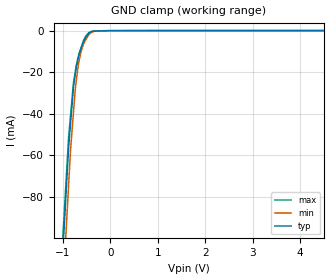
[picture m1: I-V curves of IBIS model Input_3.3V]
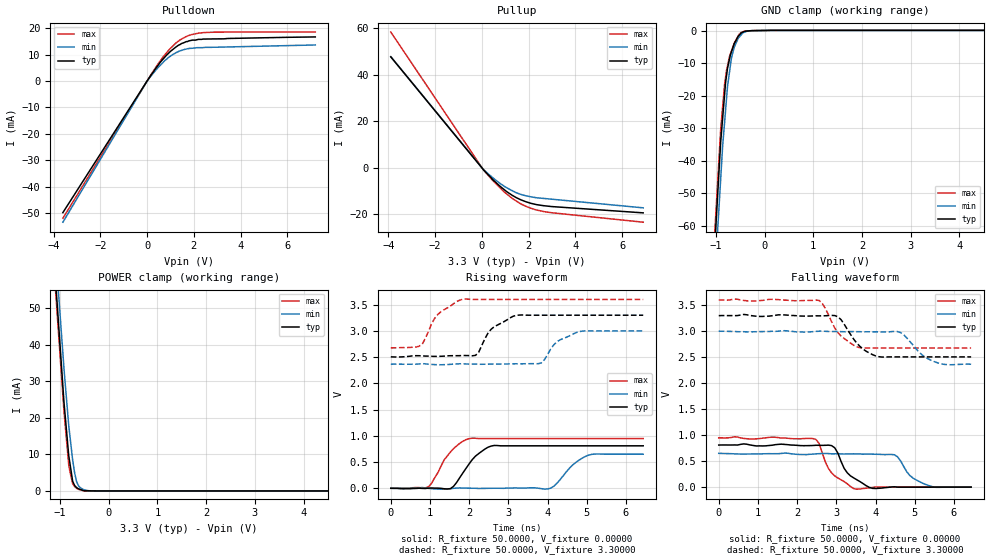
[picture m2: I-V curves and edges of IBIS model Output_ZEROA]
[IBIS Ver]   3.2
[Comment Char] |_char
[File Name]   pcm1748e.ibs
[File Rev]   3.0
[Source]
| This model file was created by Teraspeed Consulting Group LLC
| (http://www.teraspeed.com/).
[Date]   10-06-2004
[Notes]   Quality Check of this IBIS model: Model Passes IBIS Check
   Model parses into ICX IS. Simulation done with Hyperlynx.
   1. MIN TYP MAX information is based on Temprature and Voltage
   characteristics only.
[Disclaimer]
| This model is designed as an aid for customers of Texas Instruments.
| TI and its licensors and suppliers make no warranties, either expressed
| or implied, with respect to this  model, including the warranties of
| merchantability or fitness for a particular purpose.
| The model is provided solely on an "as is" basis. The entire risk as to
| its quality and performance is with the customer.
[Copyright]
| (C) Copyright 2008 Texas Instruments Incorporated. All rights reserved.
[Component] PCM1748E
[Manufacturer] TI
[Package]
| variable   typ   min   max
R_pkg  1.8006E-02  1.8006E-02  1.8006E-02
L_pkg  2.1607E-09  2.1607E-09  2.1607E-09
C_pkg  6.0021E-13  6.0021E-13  6.0021E-13
[Pin] signal_name  model_name  R_pin  L_pin C_pin
1   BCK   Input_3.3V   1.7205E-02  2.4087E-09  4.9156E-13
2   DATA   Input_3.3V   1.6401E-02  2.2962E-09  4.6861E-13
3   LRCK   Input_3.3V   1.5620E-02  2.1869E-09  4.4630E-13
4   DGND   GND   1.4866E-02  2.0812E-09  4.2474E-13
5   VDD   POWER   1.4866E-02  2.0812E-09  4.2474E-13
6   VCC   POWER   1.5620E-02  2.1869E-09  4.4630E-13
7   VoutL   NC   1.6401E-02  2.2962E-09  4.6861E-13
8   VoutR   NC   1.7205E-02  2.4087E-09  4.9156E-13
9   AGND   GND   1.7205E-02  2.4087E-09  4.9156E-13
10  Vcom   POWER   1.6401E-02  2.2962E-09  4.6861E-13
11  ZEROR/ZEROA  Output_ZEROA  1.5620E-02  2.1869E-09  4.4630E-13
12  ZEROL/NA   Input_3.3V   1.4866E-02  2.0812E-09  4.2474E-13
13  MD   Input_3.3V   1.4866E-02  2.0812E-09  4.2474E-13
14  MC   Input_3.3V   1.5620E-02  2.1869E-09  4.4630E-13
15  ML   Input_3.3V   1.6401E-02  2.2962E-09  4.6861E-13
16  SCK   Input_3.3V   1.7205E-02  2.4087E-09  4.9156E-13
| Models and submodels in the file (2): Input_3.3V (Input), Output_ZEROA (Output)
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[Model] Input_3.3V
Model_type Input
Vinl  = 800.000mV
Vinh  = 2.00000V
C_comp  2.00000pF 2.00000pF 2.00000pF
| variable   typ   min   max
[Voltage Range]   3.30000V  3.00000V  3.60000V
[POWER Clamp Reference]  3.30000V  3.00000V  3.60000V
[GND Clamp Reference]   0.00000V  0.00000V  0.00000V
[Temperature Range]   25   85   -25
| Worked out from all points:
|   GND clamp passes 1 mA (typ) near -0.45 V on its own axis
[GND Clamp]
-3.3V     -1.046A    -1.078A    -999.8mA
-881mV    -55.89mA   -73.94mA   -51.06mA
-840.9mV  -44.51mA   -57.27mA   -40.77mA
-780.3mV  -27.35mA   -39.56mA   -25.27mA
-739.7mV  -20.7mA    -27.67mA   -19.41mA
-719.4mV  -17.38mA   -23.97mA   -16.48mA
-679.1mV  -13.22mA   -16.6mA    -12.61mA
-623.4mV  -8.829mA   -10.38mA   -8.374mA
-562.1mV  -4.848mA   -6.036mA   -4.405mA
-420.8mV  -625.3uA   -1.071mA   -442.3uA
61.63mV   65.1uA     47.55uA    79.25uA
6.6V      102.1uA    79.84uA    108.8uA
[POWER Clamp]
| Voltage   I(typ)   I(min)   I(max)
-3.6V     0A         0A         0A
-3.5V     0A         0A         0A
-3.4V     0A         0A         0A
7.2V      0A         0A         0A
[Model] Output_ZEROA
Model_type Output
Vref  = 0.00000V
Cref  = 2.00000pF
Vmeas = 1.65000V
C_comp  2.00000pF 2.00000pF 2.00000pF
| variable   typ   min   max
[Voltage Range]   3.30000V  3.00000V  3.60000V
[POWER Clamp Reference]  3.30000V  3.00000V  3.60000V
[Pullup Reference]   3.30000V  3.00000V  3.60000V
[Pulldown Reference]   0.00000V  0.00000V  0.00000V
[GND Clamp Reference]   0.00000V  0.00000V  0.00000V
[Temperature Range]   25   85   -25
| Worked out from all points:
|   slope of the pulldown table from 0 to 0.495 V, typ, clamps not added: 79.2 ohm
|   slope of the pullup table from 0 to 0.495 V, typ, clamps not added: 93 ohm
|   GND clamp passes 1 mA (typ) near -0.49 V on its own axis
|   POWER clamp passes 1 mA (typ) near -0.67 V on its own axis
|   rising waveform, R_fixture 50.0000, V_fixture 0.00000: 20-80 % time 496ps typ, 493ps min, 492ps max; typ from 0 V to 0.81 V
|   falling waveform, R_fixture 50.0000, V_fixture 0.00000: 20-80 % time 435ps typ, 434ps min, 417ps max; typ from 0.81 V to 0 V
|   falling waveform, R_fixture 50.0000, V_fixture 3.30000: 20-80 % time 473ps typ, 494ps min, 464ps max; typ from 3.3 V to 2.51 V
|   rising waveform, R_fixture 50.0000, V_fixture 3.30000: 20-80 % time 511ps typ, 508ps min, 501ps max; typ from 2.51 V to 3.3 V
[GND Clamp]
-3.3V     -663.9mA   -649.4mA   -654.5mA
-901.3mV  -34.29mA   -45.71mA   -30.48mA
-861mV    -27mA      -35.59mA   -23.51mA
-820.7mV  -19.68mA   -28.2mA    -16.52mA
-800.4mV  -15.99mA   -24.47mA   -14.33mA
-760mV    -11.56mA   -17.07mA   -10.77mA
-679.1mV  -6.503mA   -8.377mA   -6.246mA
-623.5mV  -4.109mA   -5.157mA   -3.867mA
-542.3mV  -1.775mA   -2.401mA   -1.705mA
-420.8mV  -320.8uA   -560.4uA   -245.7uA
219mV     59.07uA    63.58uA    60.52uA
6.6V      59.47uA    63.58uA    67.83uA
[Pulldown]
-3.6V     -49.86mA   -53.5mA    -52mA
0V        413.4nA    -23.98uA   -32.27uA
501.5mV   6.331mA    5.407mA    6.894mA
820.4mV   9.694mA    8.204mA    10.57mA
1.139V    12.23mA    10.29mA    13.58mA
1.402V    13.81mA    11.42mA    15.55mA
1.679V    14.98mA    12.15mA    16.89mA
1.882V    15.42mA    12.42mA    17.57mA
2.422V    15.94mA    12.72mA    18.39mA
7.2V      16.74mA    13.69mA    18.58mA
[Pullup]
-3.9V     47.66mA    47.79mA    58.36mA
77.7mV    -1.111mA   -954.5uA   -1.163mA
761.3mV   -7.948mA   -6.718mA   -8.61mA
1.281V    -11.86mA   -9.89mA    -13.18mA
1.661V    -13.88mA   -11.54mA   -15.64mA
1.938V    -14.91mA   -12.28mA   -16.94mA
2.621V    -16.41mA   -13.28mA   -18.9mA
6.9V      -19.51mA   -17.35mA   -23.53mA
[POWER Clamp]
-3.3V     482.3mA    472.9mA    476.2mA
-1.12V    62.92mA    70.53mA    60.14mA
-1.059V   51.29mA    59.37mA    48.59mA
-1.019V   43.5mA     51.9mA     40.87mA
-917.8mV  24.11mA    33.29mA    21.63mA
-821.6mV  9.739mA    17.94mA    7.222mA
-740.9mV  2.661mA    8.489mA    1.999mA
-700.4mV  1.478mA    4.98mA     1.206mA
-659.8mV  903.6uA    2.513mA    708.6uA
-619.5mV  579.5uA    1.379mA    436.6uA
-381.6mV  25.51uA    2.953uA    5.591uA
6.6V      0A         0A         0A
[Rising Waveform]
R_fixture = 50.0000
V_fixture = 0.00000
V_fixture_min = 0.00000
V_fixture_max = 0.00000
0s        0V         0V         0V
960ps     1.932mV    -2.072mV   27.54mV
1.52ns    -6.905mV   -8.712mV   690.2mV
2ns       467.3mV    1.578mV    947.5mV
2.56ns    804.4mV    114.3uV    947.8mV
4ns       809.6mV    -13.09mV   947.8mV
4.24ns    809.6mV    96.46mV    947.8mV
4.64ns    809.6mV    443.7mV    947.8mV
5.04ns    809.6mV    629.9mV    947.8mV
6.44ns    809.6mV    650mV      947.8mV
[Falling Waveform]
R_fixture = 50.0000
V_fixture = 0.00000
V_fixture_min = 0.00000
V_fixture_max = 0.00000
0s        809.6mV    650mV      947.8mV
2.48ns    805.1mV    639.7mV    917.3mV
2.88ns    798.4mV    640.6mV    273.7mV
3.28ns    275.7mV    639.1mV    63.77mV
3.52ns    143.2mV    638.4mV    -39.35mV
3.92ns    -23.12mV   634.1mV    -7.117mV
4.48ns    6.278mV    622.7mV    0V
4.88ns    0V         220.8mV    0V
5.44ns    0V         10.28mV    0V
6.44ns    0V         0V         0V
[Falling Waveform]
R_fixture = 50.0000
V_fixture = 3.30000
V_fixture_min = 3.00000
V_fixture_max = 3.60000
0s        3.3V       3V         3.6V
2.56ns    3.296V     2.999V     3.592V
2.96ns    3.301V     2.994V     3.062V
3.12ns    3.223V     2.992V     2.907V
3.44ns    2.851V     2.993V     2.732V
3.76ns    2.615V     2.989V     2.677V
4.08ns    2.51V      2.987V     2.677V
4.56ns    2.506V     2.994V     2.677V
5.44ns    2.506V     2.432V     2.677V
6.44ns    2.506V     2.365V     2.677V
[Rising Waveform]
R_fixture = 50.0000
V_fixture = 3.30000
V_fixture_min = 3.00000
V_fixture_max = 3.60000
0s        2.506V     2.365V     2.677V
800ps     2.524V     2.376V     2.744V
1.2ns     2.514V     2.357V     3.314V
1.84ns    2.532V     2.373V     3.605V
2.16ns    2.534V     2.368V     3.6V
2.56ns    3.032V     2.368V     3.6V
3.2ns     3.297V     2.374V     3.6V
3.84ns    3.3V       2.39V      3.6V
4.8ns     3.3V       2.986V     3.6V
6.44ns    3.3V       3V         3.6V
[Ramp]
| variable  typ   min   max
dV/dt_r   486.043m/420.508p  389.993m/472.835p  568.328m/391.970p
dV/dt_f   481.081m/426.304p  381.533m/473.539p  555.450m/394.914p
R_load = 50.0000Ohms
